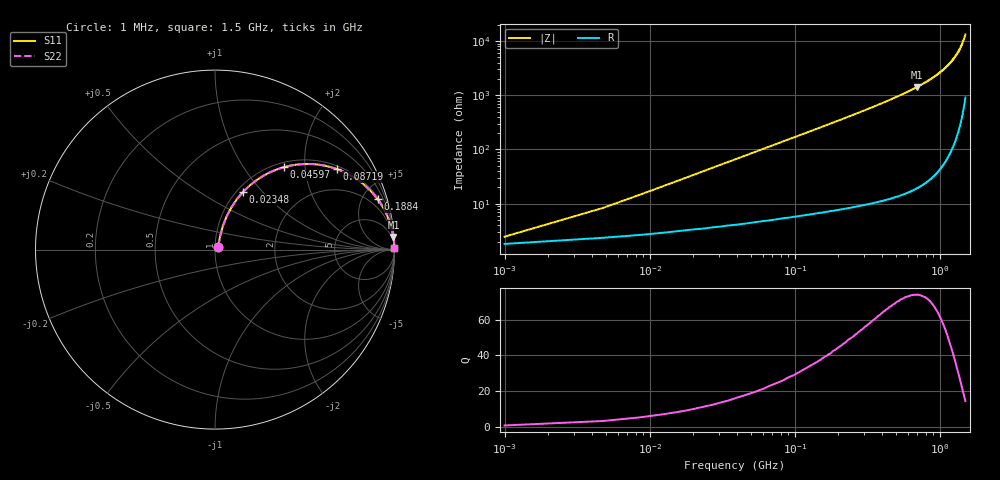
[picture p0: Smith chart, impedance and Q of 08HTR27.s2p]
! Coilcraft 0805HT-R27 Chip Inductor
! 6 August 2004
# MHZ S MA R 50
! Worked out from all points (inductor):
!   401 points, 1 MHz to 1.5 GHz, reference 50 ohm
!   read as one part in series: L = 268 nH near 8.495 MHz
!   highest Q = 73.8 at 690.5 MHz (marker M1), where L = 324 nH
!   S11 on the Smith chart (normalised r, x): 1 MHz: 1.04, +0.03; 23.48 MHz: 1.07, +0.79; 45.97 MHz: 1.09, +1.55; 87.19 MHz: 1.11, +2.95; 188.4 MHz: 1.14, +6.43; 1.5 GHz: open
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1  0.024 41.6  0.982 -0.9  0.982 -0.9  0.024 41.6
4.748  0.081 69.2  0.974 -4.5  0.974 -4.5  0.081 69.2
12.243  0.198 70.6  0.953 -11.3  0.953 -11.3  0.198 70.6
15.99  0.254 68.7  0.938 -14.6  0.938 -14.6  0.254 68.7
23.485  0.358 64.0  0.903 -20.9  0.903 -20.9  0.358 64.0
34.727  0.492 56.8  0.838 -29.4  0.838 -29.4  0.492 56.8
45.97  0.597 50.2  0.77 -36.6  0.77 -36.6  0.597 50.2
64.708  0.722 41.3  0.661 -46.1  0.661 -46.1  0.722 41.3
87.193  0.814 33.5  0.552 -54.4  0.552 -54.4  0.814 33.5
105.93  0.861 28.7  0.481 -59.4  0.481 -59.4  0.861 28.7
128.415  0.899 24.4  0.413 -63.9  0.413 -63.9  0.899 24.4
188.375  0.949 17.2  0.295 -71.5  0.295 -71.5  0.949 17.2
252.083  0.97 12.9  0.223 -76.0  0.223 -76.0  0.97 12.9
360.76  0.985 8.9  0.155 -80.2  0.155 -80.2  0.985 8.9
503.165  0.993 6.1  0.106 -83.1  0.106 -83.1  0.993 6.1
690.54  0.997 4.1  0.071 -85.2  0.071 -85.2  0.997 4.1
750.5  0.997 3.6  0.063 -85.6  0.063 -85.6  0.997 3.6
1001.582  0.999 2.2  0.038 -86.9  0.038 -86.9  0.999 2.2
1102.765  0.999 1.7  0.03 -87.2  0.03 -87.2  0.999 1.7
1252.665  0.999 1.2  0.021 -87.4  0.021 -87.4  0.999 1.2
1391.322  0.999 0.7  0.013 -87.0  0.013 -87.0  0.999 0.7
1500  0.999 0.4  0.00756 -85.6  0.00756 -85.6  0.999 0.4
